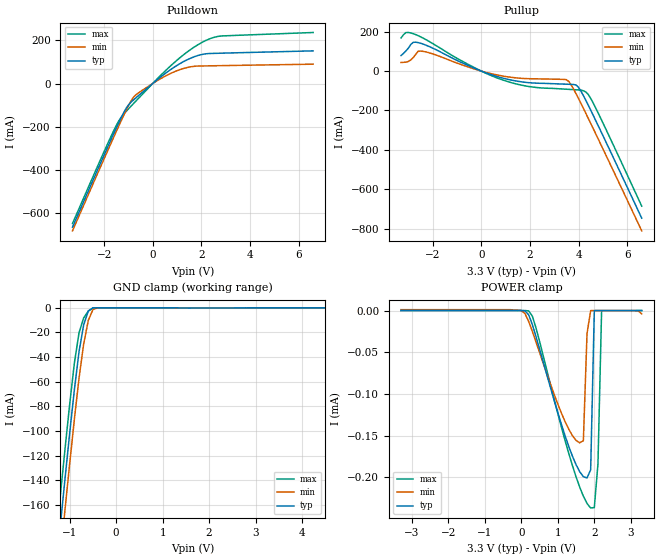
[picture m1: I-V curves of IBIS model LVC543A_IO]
|TEXAS INSTRUMENTS INCORPORATED
|Standard Linear and Logic Group
|IBIS Model of LVC543A
|Octal Registered Transceiver with 3-State Outputs
|SSOP 24-pin (DB), SOP 24-pin (DW), TSSOP 24-pin (PW) Package
[IBIS Ver]   2.1
[Comment char]  |_char
[File Name]   lvc543a.ibs
[File Rev]   1.0
[Date]   10/20/97
[Source]   File originated at Texas Instruments, Inc.
[Notes]   The following is an IBIS list for the LVC543A.
|   - All test data contained in this file are derived from
|   hspice(tm) simulations.
|   - File created by Ramzi Ammar, SLL Applications
|   - This file may be incomplete or may not be fully compliant
|   with the IBIS specification. It will be replaced with a
|   version that is IBIS Revision 3.2 compliant and is complete
|   and accurate.
|   Please email all questions and comments to sllibis@ti.com.
[Disclaimer] Property of Texas Instruments Incorporated.  Unauthorized
   reproduction and/or distribution is strictly prohibited.
   This product is protected under copyright law.
   Created 1997, (C) Copyright 1997, Texas Instruments Inc.,
   All Rights Reserved
   UNLESS THERE IS A SIGNED, WRITTEN AGREEMENT TO THE
   CONTRARY, TEXAS INSTRUMENTS ("TI") IS PROVIDING THE IBIS
   MODELS "AS IS" AND WITHOUT ANY WARRANTY, EXPRESSED OR
   IMPLIED.  TI assumes no liability for:
   1) the accuracy of the IBIS models provided to your
   company;
   2) the proper functioning of these IBIS models in your
   design or for any resulting applications; or
   3) infringement of patents, copyrights or intellectual
   property rights resulting from your use of these IBIS
   models.
   TI provides IBIS Models as a service to our customers.
   You and your company shall not distribute, sell or give
   these models to anyone else without prior written
   permission from TI.
   TI reserves the right to make changes to our products or
   to discontinue any semiconductor product or service
   without notice, and advises our customers to obtain the
   latest version of relevant information to verify, before
   placing orders, that the information being relied on is
   current.
   Please be aware that your receipt and use of the IBIS
   information provided shall serve as acceptance of these
   terms and conditions.  If you do not accept these terms,
   you should return or destroy the IBIS models and any
   other accompanying information immediately.
[Component]   LVC543A_DB
[Manufacturer]  Texas Instruments, Inc.
[Package]
|	  typ 	min   max
R_pkg	  0.045	0.04   0.049
L_pkg	  3.668nH	3.226nH	4.415nH
C_pkg	  0.416pF	0.349pF	0.507pF
[Pin]	signal_name	model_name	 R_pin	L_pin   C_pin
1   LEBA	NC   0.042	4.299nH	0.503pF
2   OEBA	NC   0.04   3.96nH	0.499pF
3   A1	LVC543A_IO	 0.042	3.775nH	0.417pF
4   A2	LVC543A_IO	 0.047	3.487nH	0.369pF
5   A3   LVC543A_IO	 0.046	3.347nH	0.352pF
6   A4	LVC543A_IO	 0.049	3.352nH	0.371pF
7   A5	LVC543A_IO	 0.046	3.226nH	0.363pF
8   A6	LVC543A_IO	 0.047	3.289nH	0.349pF
9   A7	LVC543A_IO	 0.047	3.347nH	0.361pF
10   A8	LVC543A_IO	 0.041	3.576nH	0.409pF
11   CEAB	NC   0.041	3.995nH	0.503pF
12   GND	GND   0.045	4.415nH	0.507pF
13   OEAB	NC   0.043	4.337nH	0.506pF
14   LEAB	NC   0.042	4.003nH	0.504pF
15   B8	LVC543A_IO   0.041	3.686nH	0.41pF
16   B7	LVC543A_IO	 0.048	3.355nH	0.349pF
17   B6	LVC543A_IO	 0.047	3.301nH	0.353pF
18   B5	LVC543A_IO	 0.048	3.268nH	0.366pF
19   B4	LVC543A_IO	 0.048	3.269nH	0.366pF
20   B3	LVC543A_IO	 0.047	3.314nH	0.349pF
21   B2	LVC543A_IO	 0.048	3.399nH	0.355pF
22   B1	LVC543A_IO	 0.041	3.688nH	0.412pF
23   CEBA	NC   0.042	4.003nH	0.504pF
24   VCC	POWER   0.043	4.347nH	0.505pF
|   Component LVC543A_DW
[Component]   LVC543A_DW
[Manufacturer]  Texas Instruments, Inc.
[Package]
|   typ   min   max
R_pkg   0.037	0.03   0.047
L_pkg   5.146nH  3.993nH	6.885nH
C_pkg   0.758pF  0.512pF	1.067pF
[Pin]	signal_name	model_name	 R_pin	L_pin   C_pin
1   LEBA	NC   0.039	6.885nH	1.067pF
2   OEBA	NC   0.042	5.95nH	0.958pF
3   A1	LVC543A_IO	 0.047	5.317nH	0.791pF
4   A2	LVC543A_IO	 0.031	4.651nH	0.611pF
5   A3	LVC543A_IO	 0.03   3.993nH	0.512pF
6   A4	LVC543A_IO	 0.03   4.083nH	0.611pF
7   A5	LVC543A_IO	 0.03   4.083nH	0.611pF
8   A6	LVC543A_IO	 0.03   3.993nH	0.512pF
9   A7	LVC543A_IO   0.031	4.652nH	0.611pF
10   A8	LVC543A_IO   0.047	5.317nH	0.791pF
11   CEAB	NC   0.042	5.95nH	0.959pF
12   GND	GND   0.039	6.885nH	1.067pF
13   OEAB	NC   0.039	6.885nH	1.067pF
14   LEAB	NC   0.042	5.95nH	0.959pF
15   B8	LVC543A_IO   0.047	5.317nH	0.791pF
16   B7	LVC543A_IO	 0.031	4.652nH	0.611pF
17   B6	LVC543A_IO	 0.03   3.993nH	0.512pF
18   B5	LVC543A_IO	 0.03   4.083nH	0.61pF
19   B4	LVC543A_IO	 0.03   4.083nH	0.61pF
20   B3	LVC543A_IO	 0.03   3.993nH	0.512pF
21   B2	LVC543A_IO	 0.031	4.651nH	0.611pF
22   B1	LVC543A_IO	 0.047	5.317nH	0.791pF
23   CEBA	NC   0.042	5.95nH	0.958pF
24   VCC	POWER   0.039	6.885nH	1.067pF
|   Component LVC543A_PW
[Component]   LVC543A_PW
[Manufacturer]  Texas Instruments, Inc.
[Package]
|		typ   min	max
R_pkg		0.039   0.03	0.046
L_pkg		2.685nH  2.367nH	3.177nH
C_pkg		0.32pF   0.252pF	0.434pF
[Pin]	signal_name	model_name	 R_pin 	L_pin   C_pin
1   LEBA	LVC543A_IO	 0.037	3.153nH	0.434pF
2   OEBA	LVC543A_IO	 0.034	2.629nH	0.341pF
3   A1	LVC543A_IO	 0.032	2.86nH	0.347pF
4   A2	LVC543A_IO	 0.042	2.741nH	0.29pF
5   A3   LVC543A_IO	 0.046	2.6nH   0.262pF
6   A4	LVC543A_IO	 0.043	2.414nH	0.266pF
7   A5	LVC543A_IO	 0.042	2.367nH	0.262pF
8   A6   LVC543A_IO	 0.044	2.461nH	0.252pF
9   A7	LVC543A_IO   0.042	2.543nH	0.274pF
10   A8	LVC543A_IO   0.03   2.616nH	0.332pF
11   CEAB	NC   0.037	2.67nH	0.346pF
12   GND	GND   0.039	3.177nH	0.433pF
13   OEAB	NC   0.037	3.111nH	0.431pF
14   LEAB	NC   0.037	2.656nH	0.345pF
15   B8	LVC543A_IO   0.031	2.739nH	0.34pF
16   B7	LVC543A_IO	 0.042	2.649nH	0.282pF
17   B6	LVC543A_IO	 0.046	2.532nH	0.257pF
18   B5	LVC543A_IO	 0.044	2.425nH	0.266pF
19   B4	LVC543A_IO	 0.044	2.425nH	0.266pF
20   B3	LVC543A_IO	 0.046	2.532nH	0.257pF
21   B2	LVC543A_IO	 0.042	2.648nH	0.282pF
22   B1	LVC543A_IO	 0.031	2.738nH	0.339pF
23   CEBA	NC   0.036	2.653nH	0.344pF
24   VCC	POWER   0.037	3.11nH	0.431pF
| Models and submodels in the file (1): LVC543A_IO (I/O)
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|   Model LVC543A_IO
[Model]   LVC543A_IO
Model_type   I/O
Polarity   Inverting
Enable   Active-Low
Vinl = 0.8V
Vinh = 2.0V
|variable   typ   min   max
C_comp   7.5pF   NA   NA
[Voltage range]   3.3   3.0   3.6
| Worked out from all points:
|   slope of the pulldown table from 0 to 0.495 V, typ, clamps not added: 11 ohm
|   slope of the pullup table from 0 to 0.495 V, typ, clamps not added: 22.7 ohm
|   GND clamp passes 1 mA (typ) near -0.54 V on its own axis
[Pullup]   | Note: Vtable = Vcc - Voutput
|   Voltage   I(typ)   I(min)   I(max)
-3.3V     79.04mA    43.89mA    168.3mA
-3.1V     101.9mA    45.6mA     195.6mA
-2.8V     146.2mA    68.19mA    190mA
-2.6V     144.7mA    100.6mA    180.1mA
-500mV    26.15mA    19.43mA    31.51mA
800mV     -32.95mA   -23.32mA   -41.57mA
2V        -59.23mA   -38.84mA   -79.22mA
3.5V      -66.61mA   -43.71mA   -92.1mA
3.7V      -67.54mA   -70.64mA   -93.57mA
4V        -82.56mA   -139.7mA   -95.77mA
4.4V      -173.1mA   -239.8mA   -118.5mA
6.6V      -747.2mA   -811.6mA   -686mA
[Pulldown]
|   Voltage   I(typ)   I(min)   I(max)
-3.3V     -667.5mA   -684.7mA   -650.8mA
-1.5V     -207.3mA   -223.3mA   -195.4mA
-1.3V     -159.4mA   -173.9mA   -157.3mA
-1.1V     -116.6mA   -126.1mA   -130.4mA
-800mV    -77.43mA   -65.31mA   -94.48mA
-600mV    -57.81mA   -44.52mA   -70.78mA
400mV     36.73mA    27.26mA    45.85mA
1.1V      91mA       63.71mA    117.9mA
1.8V      127.9mA    80.82mA    176mA
2.4V      139.6mA    82.23mA    210.1mA
2.9V      141.1mA    83.21mA    221.3mA
6.6V      151.7mA    89.79mA    237mA
[GND_Clamp]
|   Voltage   I(typ)   I(min)   I(max)
-3.3V     -1.009A    -1.033A    -985.8mA
-1.3V     -214.2mA   -239.3mA   -189.7mA
-1.2V     -175.9mA   -201mA     -151.5mA
-1.1V     -138.2mA   -163.3mA   -114mA
-1V       -101.5mA   -126.2mA   -77.91mA
-900mV    -66.49mA   -90.46mA   -44.84mA
-800mV    -35.67mA   -57.14mA   -20.29mA
-700mV    -13.84mA   -29.32mA   -8.191mA
-600mV    -2.515mA   -10.19mA   -2.697mA
-500mV    -71.34uA   -1.341mA   -142.5uA
-300mV    -90.6nA    -4.019uA   -513nA
6.6V      45.46nA    1.093uA    15.11nA
[POWER_Clamp]   | Note: Vtable = Vcc - Voutput
|   Voltage   I(typ)   I(min)   I(max)
-3.3V     45.46nA    1.092uA    15.8nA
-100mV    16.6nA     426.1nA    9.053nA
200mV     -5.058uA   -13.02uA   -398.5nA
1.1V      -136.8uA   -123.2uA   -140.1uA
1.6V      -193.2uA   -158.6uA   -211.8uA
1.7V      -199.1uA   -156uA     -222.6uA
1.8V      -200.7uA   -27.73uA   -231.2uA
1.9V      -190.9uA   -3.627nA   -236.7uA
2V        -4.778nA   -4.02nA    -236.2uA
2.1V      -2.779nA   -4.424nA   -183.9uA
2.2V      -3.066nA   -4.828nA   -21.34nA
3.3V      -6.227nA   -4.019uA   -5.96nA
[Ramp]
|Variable   typ   min   max
dV/dt_r   1.2882E+00/6.0154E-10  9.9503E-01/8.9713E-10  1.5303E+00/4.2925E-10
dV/dt_f   1.6231E+00/3.0064E-09  1.3745E+00/7.6610E-09  1.8424E+00/1.7254E-09
